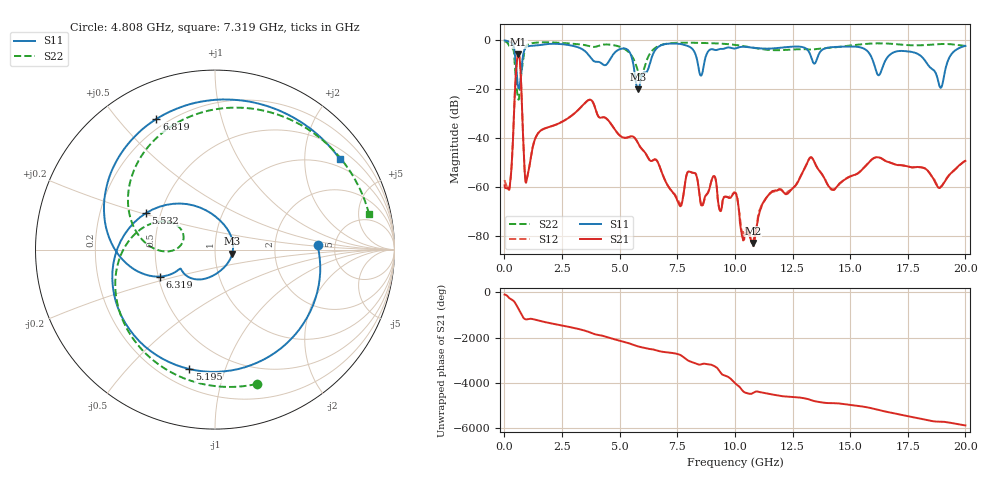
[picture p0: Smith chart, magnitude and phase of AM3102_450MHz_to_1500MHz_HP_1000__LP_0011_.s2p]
!Agilent Technologies,E8364B,MY43040894,A.07.50.67
!Agilent E8364B: A.07.50.67
!Date: Thursday, January 11, 2018 05:56:58
!Correction: S11(Full 2 Port(1,2))
!S21(Full 2 Port(1,2))
!S12(Full 2 Port(1,2))
!S22(Full 2 Port(1,2))
!S2P File: Measurements: S11, S21, S12, S22:
# Hz S  dB  R 50
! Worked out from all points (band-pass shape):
!   1601 points, 10 MHz to 20 GHz, reference 50 ohm
!   highest |S21| = -5.78 dB at 609.7 MHz (marker M1); lowest = -83.0 dB at 10.79 GHz (marker M2)
!   |S21| within 3 dB of the highest: 541.6 MHz to 676.1 MHz (134.5 MHz wide, 22.1 % of centre)
!   lowest |S11| = -20.1 dB at 5.795 GHz (marker M3), VSWR 1.22, Z = 60.5 - j2.81 ohm
!   |S11| at or under -10 dB: 5.597 GHz to 6.299 GHz (702.2 MHz wide, 11.8 % of centre); 16.05 GHz to 16.45 GHz (401.2 MHz wide, 2.47 % of centre); 18.37 GHz to 19.18 GHz (812.4 MHz wide, 4.33 % of centre)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
!   |S22| runs from -24.3 to -0.4 dB; largest |S21 - S12| = 0.0019
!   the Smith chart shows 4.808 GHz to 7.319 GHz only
!   S11 on the Smith chart (normalised r, x): 4.808 GHz: 3.65, +0.26; 5.195 GHz: 0.31, -0.76; 5.532 GHz: 0.41, +0.21; 6.319 GHz: 0.51, -0.17; 6.819 GHz: 0.16, +0.64; 7.319 GHz: 0.76, +2.92
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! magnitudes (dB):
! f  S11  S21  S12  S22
! 10 MHz  -0.1  -59.4  -57.2  -0.4
! 259.9 MHz  -0.8  -57.6  -57.9  -2.8
! 609.7 MHz  -19.5  -5.8  -5.8  -24.3
! 972 MHz  -2.6  -57.1  -57.0  -2.1
! 1.484 GHz  -2.0  -37.8  -37.8  -0.9
! 3.346 GHz  -3.5  -27.1  -27.1  -1.8
! 4.808 GHz  -4.9  -36.8  -36.8  -2.1
! 5.195 GHz  -3.3  -39.9  -39.9  -3.4
! 5.532 GHz  -7.2  -39.3  -39.3  -6.5
! 5.795 GHz  -20.1  -42.1  -42.1  -12.6
! 6.319 GHz  -9.3  -49.3  -49.3  -5.4
! 6.682 GHz  -2.7  -50.5  -50.5  -2.4
! 6.819 GHz  -2.0  -53.9  -53.9  -1.9
! 7.319 GHz  -1.3  -62.5  -62.5  -1.1
! 8.531 GHz  -14.5  -67.0  -67.6  -1.1
! 10.01 GHz  -3.4  -62.5  -62.4  -1.9
! 10.79 GHz  -3.0  -83.0  -83.8  -3.0
! 13.34 GHz  -7.8  -48.1  -48.1  -3.8
! 14.24 GHz  -2.8  -61.2  -61.2  -3.0
! 16.68 GHz  -6.3  -49.9  -49.9  -1.4
! 18.93 GHz  -19.5  -60.1  -60.0  -1.5
! 20 GHz  -2.3  -49.4  -49.4  -2.3
